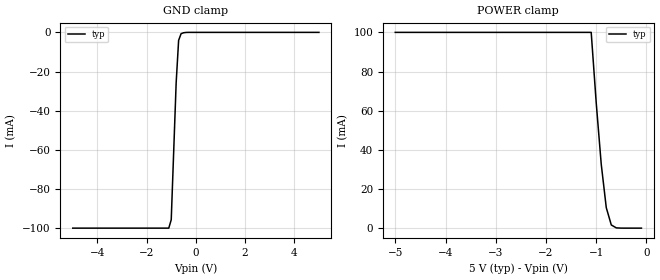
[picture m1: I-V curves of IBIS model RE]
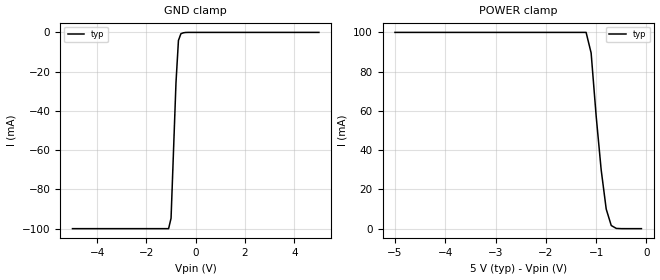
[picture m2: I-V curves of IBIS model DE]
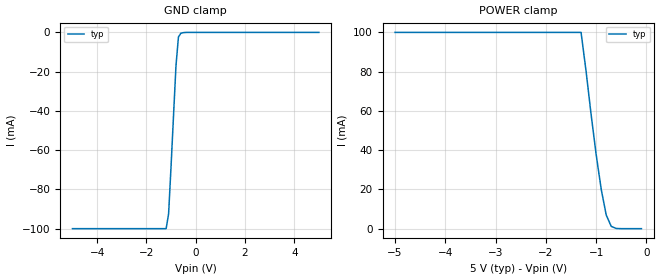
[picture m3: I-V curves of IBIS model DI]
| IBIS file 487.ibs created at Maxim Integrated Products
[IBIS ver]   2.1
[File name]   487.ibs
[File Rev]   1.0
[Date]   December 05, 2002
[Source]   Rise and fall ramps, and IV curves were taken on the bench
   using an Oscilloscope and Semiconductor Parameter Analyzer.
[Notes]   This is a Low-Power Slew-Rate-Limited RS422 Transceiver.
[Disclaimer] Maxim Integrated Products hereby grants the user of this
   IBIS model a non-exclusive, nontransferable license to
   use this IBIS model under the following terms. Before
   using this IBIS model, the user should read this license.
   If the user does not accept these terms, the IBIS model
   should be returned to Maxim Integrated Products within 30
   days. The user is granted this license only to use the
   IBIS model and is not granted rights to sell, load, rent,
   lease or license the IBIS model in whole or in part, or
   in modified form to anyone other than user. User may modify
   the IBIS model to suit its specific applications but rights
   to derivative works and such modifications shall belong to
   Maxim Integrated Products. This IBIS model is provided on
   an "AS IS" basis and Maxim Integrated Products makes
   absolutely no warranty with respect to the information
   contained herein. MAXIM INTEGRATED PRODUCTS DISCLAIMS AND
   CUSTOMER WAIVES ALL WARRANTIES, EXPRESS OR IMPLIED,
   INCLUDING WARRANTIES OF MERCHANTABILITY OR FITNESS FOR A
   PARTICULAR PURPOSE. The entire risk as to quality and
   performance is with the Customer. ACCORDINGLY, IN NO EVENT
   SHALL THE COMPANY BE LIABLE FOR ANY DAMAGES, WHETHER IN
   CONTRACT OR TORT, INCLUDING ANY LOST PROFITS OR OTHER
   INCIDENTAL, CONSEQUENTIAL, EXEMPLARY, OR PUNITIVE DAMAGES
   ARISING OUT OF THE USE OR APPLICATION OF THE IBIS model
   provided in this package.Further, Maxim Integrated Products
   reserves the right to make changes without notice to any
   product herein to improve reliability, function, or design.
   Maxim Integrated Products does not convey any license under
   patent rights or any other intellectual property rights,
   including those of third parties. Maxim Integrated Products
   is not obligated to provide maintenance or support for the
   licensed IBIS model.
[Copyright]   COPYRIGHT MAXIM INTEGRATED PRODUCTS 2002 ALL RIGHTS PRESERVE.
|   Component MAX487
[Component]   MAX487
[Manufacturer]   Maxim Integrated Products
[Package]
| variable   typ   min   max
R_pkg   55.5m   NA   NA
L_pkg   1.57nH   NA   NA
C_pkg   0.252pF   NA   NA
[Pin]  signal_name   model_name   R_pin   L_pin   C_pin
1   RO   RO
2   REB   RE
3   DE   DE
4   DI   DI
5   GND   GND
6   A   Driver_IO
7   B   Driver_IO
8   VCC   POWER
| Models and submodels in the file (5): RE (Input), DE (Input), DI (Input), RO (3-state), Driver_IO (I/O)
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|   Driver Output Receiver Enable
[Model]   RE
|Signals   REB
Model_type   Input
Enable   Active-Low
Vinl = 0.8V
Vinh = 2.0V
C_comp   0.538pF   NA   NA
[Temperature Range]   25   -40   85
[Voltage Range]   5.00V   4.75V   5.25V
[POWER Clamp Reference]   5.00V   4.75V   5.25V
[GND Clamp Reference]   0.00V   0.00V   0.00V
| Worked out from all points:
|   GND clamp passes 1 mA (typ) near -0.61 V on its own axis
|   POWER clamp passes 1 mA (typ) near -0.66 V on its own axis
[POWER_clamp]
| Note that the[POWER_clamp]voltage table is referenced to Vcc
| and is calculated using Vtable=Vcc - Vmeasured.
| Also, the Semiconductor Parameter Analyzer (Force and Sense)
| clamps the supply current to 100mA to protect the system.
| V(V)  I(typ)   I(min)  I(max)
-5V       100mA      NA         NA
-1.1V     100mA      NA         NA
-1V       63.98mA    NA         NA
-900mV    32.61mA    NA         NA
-800mV    10.47mA    NA         NA
-700mV    1.616mA    NA         NA
-600mV    127.9uA    NA         NA
-500mV    5.943uA    NA         NA
-400mV    152.8nA    NA         NA
-300mV    3.501nA    NA         NA
-200mV    101pA      NA         NA
-100mV    0A         NA         NA
[GND_clamp]
| Note that the[GND_clamp]voltage table is referenced to Gnd.
| Also, the Semiconductor Parameter Analyzer (Force and Sense)
| clamps the supply current to 100mA to protect the system.
| V(V)  I(typ)   I(min)  I(max)
-5V       -100mA     NA         NA
-1.1V     -100mA     NA         NA
-1V       -95.72mA   NA         NA
-800mV    -25.82mA   NA         NA
-700mV    -4.099mA   NA         NA
-600mV    -674.2uA   NA         NA
-300mV    -1.653uA   NA         NA
5V        0A         NA         NA
|   Driver Output Transmitter Enable
[Model]   DE
|Signals   DE
Model_type   Input
Enable   Active-High
Vinl = 0.8V
Vinh = 2.0V
C_comp   0.538pF   NA   NA
[Temperature Range]   25   -40   85
[Voltage Range]   5.00V   4.75V   5.25V
[POWER Clamp Reference]   5.00V   4.75V   5.25V
[GND Clamp Reference]   0.00V   0.00V   0.00V
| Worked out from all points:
|   GND clamp passes 1 mA (typ) near -0.61 V on its own axis
|   POWER clamp passes 1 mA (typ) near -0.66 V on its own axis
[POWER_clamp]
| Note that the[POWER_clamp]voltage table is referenced to Vcc
| and is calculated using Vtable=Vcc - Vmeasured.
| Also, the Semiconductor Parameter Analyzer (Force and Sense)
| clamps the supply current to 100mA to protect the system.
| V(V)  I(typ)   I(min)  I(max)
-5V       100mA      NA         NA
-1.2V     100mA      NA         NA
-1.1V     89.52mA    NA         NA
-1V       57.35mA    NA         NA
-900mV    29.9mA     NA         NA
-800mV    9.953mA    NA         NA
-700mV    1.601mA    NA         NA
-600mV    127.9uA    NA         NA
-100mV    0A         NA         NA
[GND_clamp]
| Note that the[GND_clamp]voltage table is referenced to Gnd.
| Also, the Semiconductor Parameter Analyzer (Force and Sense)
| clamps the supply current to 100mA to protect the system.
| V(V)  I(typ)   I(min)  I(max)
-5V       -100mA     NA         NA
-1.1V     -100mA     NA         NA
-1V       -94.71mA   NA         NA
-800mV    -25.58mA   NA         NA
-700mV    -4.085mA   NA         NA
-600mV    -672.1uA   NA         NA
-300mV    -1.656uA   NA         NA
5V        0A         NA         NA
|   Driver Transmitter Input
[Model]   DI
|Signals   DI
Model_type   Input
Enable   Active-High
Vinl = 0.8V
Vinh = 2.0V
C_comp   0.538pF   NA   NA
[Temperature Range]   25   -40   85
[Voltage Range]   5.00V   4.75V   5.25V
[POWER Clamp Reference]   5.00V   4.75V   5.25V
[GND Clamp Reference]   0.00V   0.00V   0.00V
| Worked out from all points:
|   GND clamp passes 1 mA (typ) near -0.63 V on its own axis
|   POWER clamp passes 1 mA (typ) near -0.68 V on its own axis
[POWER_clamp]
| Note that the[POWER_clamp]voltage table is referenced to Vcc
| and is calculated using Vtable=Vcc - Vmeasured.
| Also, the Semiconductor Parameter Analyzer (Force and Sense)
| clamps the supply current to 100mA to protect the system.
| V(V)  I(typ)   I(min)  I(max)
-5V       100mA      NA         NA
-1.3V     100mA      NA         NA
-1.2V     80.08mA    NA         NA
-1.1V     58.07mA    NA         NA
-1V       37.81mA    NA         NA
-900mV    20.13mA    NA         NA
-800mV    6.95mA     NA         NA
-700mV    1.169mA    NA         NA
-600mV    91.81uA    NA         NA
-100mV    0A         NA         NA
[GND_clamp]
| Note that the[GND_clamp]voltage table is referenced to Gnd.
| Also, the Semiconductor Parameter Analyzer (Force and Sense)
| clamps the supply current to 100mA to protect the system.
| V(V)  I(typ)   I(min)  I(max)
-5V       -100mA     NA         NA
-1.2V     -100mA     NA         NA
-1.1V     -92.51mA   NA         NA
-1V       -68.24mA   NA         NA
-800mV    -16.91mA   NA         NA
-700mV    -2.348mA   NA         NA
-600mV    -385.6uA   NA         NA
-300mV    -924.4nA   NA         NA
5V        0A         NA         NA
